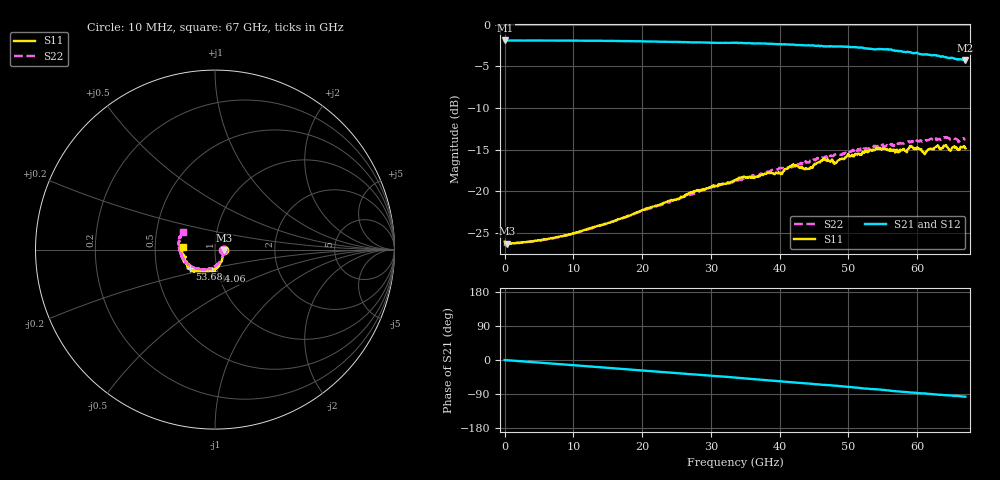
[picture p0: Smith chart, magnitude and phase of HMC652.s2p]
! Hittite Microwave Corporation
! 2 Elizabeth Drive
! Chelmsford, MA 01824
! http://www.hittite.com
! Tel: 978-250-3343
! Fax: 978-250-3373
! Device:  HMC652
! Description:  2 dB Wideband Fixed Attenuator
! Frequency:  DC - 50.00 GHz
! Package:  Die
! Ports:  2
!  Pad 1 = RF1  = Port 1
!  Pad 2 = RF2  = Port 2
! Data:  The device was measured using G-S-G Probes at the chip ports.
!  Data was collected using an calibrated network analyzer.
!  The reference plane is the pads on the chip.
! Misc:  Application 20120128
!  HMC652 Part 3
! Date Measured:  2012-07-05
! Date:  2012-07-06 MJV
! Note:
!  Hittite supplies this data as a sample of measured data at the die pads.
!  Your particular data for this product may vary.
!  Data was taken at 25 degrees C.
!  Hittite reserves the right to change this data at anytime.
# GHZ S DB R 50.0
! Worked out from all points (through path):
!   670 points, 10 MHz to 67 GHz, reference 50 ohm
!   highest |S21| = -1.90 dB at 110.1 MHz (marker M1); lowest = -4.3 dB at 67 GHz (marker M2)
!   group delay of S21, straight-line fit = 4.04 ps
!   lowest |S11| = -26.3 dB at 410.5 MHz (marker M3), VSWR 1.10, Z = 55.1 - j0.144 ohm
!   |S11| at or under -10 dB: start of sweep to end of sweep
!   |S22| runs from -26.6 to -13.5 dB; largest |S21 - S12| = 0.014
!   S11 on the Smith chart (normalised r, x): 10 MHz: 1.10, -0.00; 34.06 GHz: 0.94, -0.23; 53.68 GHz: 0.74, -0.16; 67 GHz: 0.69, +0.02
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0.01  -26.06 -0.3  -1.94 -0.1  -1.88 0.6  -26.60 -1.0
0.110135  -26.30 -0.6  -1.90 -0.2  -1.90 -0.1  -26.34 -0.5
0.410538  -26.31 -1.5  -1.91 -0.6  -1.91 -0.5  -26.31 -1.9
6.41861  -25.70 -23.8  -1.91 -8.8  -1.91 -8.7  -25.76 -27.3
11.22507  -24.77 -39.5  -1.92 -15.4  -1.93 -15.4  -24.80 -45.4
22.44014  -21.66 -69.0  -2.04 -31.1  -2.04 -31.0  -21.71 -80.3
33.55507  -18.66 -96.2  -2.18 -46.4  -2.18 -46.5  -18.68 -109.4
34.05574  -18.41 -96.8  -2.20 -47.2  -2.18 -47.3  -18.68 -110.9
40.06381  -17.88 -109.3  -2.37 -56.2  -2.34 -56.5  -17.20 -124.8
42.0665  -16.87 -115.1  -2.41 -59.3  -2.44 -59.5  -16.99 -130.9
43.76879  -17.24 -117.7  -2.47 -61.7  -2.52 -61.9  -16.39 -135.1
44.67  -17.19 -121.9  -2.49 -62.9  -2.57 -63.3  -16.40 -137.1
46.27215  -16.18 -121.7  -2.58 -65.7  -2.66 -65.6  -15.97 -141.9
48.07457  -16.68 -128.5  -2.63 -67.8  -2.71 -67.7  -15.61 -147.1
49.877  -15.66 -131.4  -2.66 -70.9  -2.73 -70.5  -15.33 -150.8
53.68211  -15.10 -143.3  -2.95 -76.9  -2.92 -76.5  -14.53 -163.2
55.88507  -15.08 -149.4  -2.96 -80.4  -2.94 -80.2  -14.44 -169.4
58.48857  -15.33 -156.6  -3.28 -84.3  -3.19 -84.1  -14.10 -178.2
59.18951  -14.70 -160.1  -3.39 -86.0  -3.31 -85.6  -14.10 179.3
60.99193  -15.41 -165.8  -3.60 -88.2  -3.48 -87.8  -13.97 173.1
62.79435  -14.62 -169.7  -3.67 -91.0  -3.59 -90.9  -13.85 166.6
67  -14.85 174.9  -4.30 -96.8  -4.17 -96.5  -13.81 150.7
